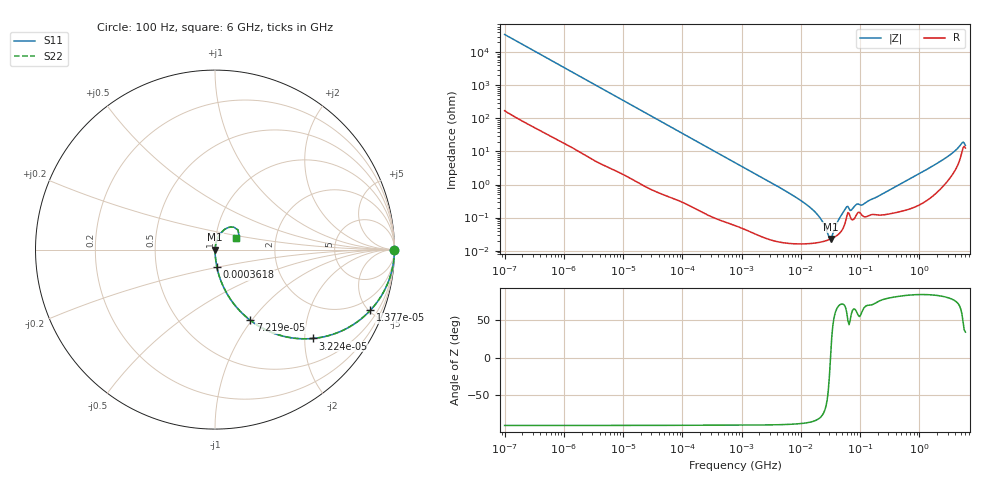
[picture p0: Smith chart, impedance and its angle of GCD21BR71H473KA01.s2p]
!Murata Part Number: GCD21BR71H473KA01
!These Parameters are Measured in Series Mode Connection
!Data Generated on Jan 08, 2026
!  o--ll--o
!Port1  Port2
!  o------o
!Operation Temp=25[degC], DC Bias Voltage=0[V]
!Freq. Start=100[Hz] Stop=6[GHz] 401[Steps]
# Hz S RI R 50
!Freq.(Hz) S11(Real) S11(Imag) S21(Real) S21(Imag) S12(Real) S12(Imag) S22(Real) S22(Imag)
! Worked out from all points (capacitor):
!   401 points, 100 Hz to 6 GHz, reference 50 ohm
!   read as one part in series: C = 45.8 nF near 109 Hz
!   lowest |Z| = 22.4 mohm at 31.85 MHz (marker M1)
!   series resonance near 31.67 MHz, so ESL is about 550 pH
!   S11 on the Smith chart (normalised r, x): 100 Hz: open; 13.77 kHz: 1.03, -5.12; 32.24 kHz: 1.01, -2.19; 72.19 kHz: 1.01, -0.98; 361.8 kHz: 1.00, -0.20; 6 GHz: 1.25, +0.17
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100  1 -0.00288  2.25e-05 0.00288  2.25e-05 0.00288  1 -0.00288
2008  0.9964 -0.0571  0.00356 0.0571  0.00356 0.0571  0.9964 -0.0571
13772  0.8662 -0.3376  0.1338 0.3376  0.1338 0.3376  0.8662 -0.3376
32244  0.5457 -0.4949  0.4543 0.4949  0.4543 0.4949  0.5457 -0.4949
40335  0.4352 -0.4926  0.5648 0.4926  0.5648 0.4926  0.4352 -0.4926
72189  0.1962 -0.3934  0.8038 0.3934  0.8038 0.3934  0.1962 -0.3934
141303  0.0615 -0.2359  0.9385 0.2359  0.9385 0.2359  0.0615 -0.2359
361830  0.0106 -0.0977  0.9894 0.0977  0.9894 0.0977  0.0106 -0.0977
774597  0.00271 -0.0462  0.9973 0.0462  0.9973 0.0462  0.00271 -0.0462
6644369  0.000191 -0.00523  0.9998 0.00523  0.9998 0.00523  0.000191 -0.00523
1.555665e7  0.000169 -0.00178  0.9998 0.00178  0.9998 0.00178  0.000169 -0.00178
2.128304e7  0.000181 -0.000947  0.9998 0.000947  0.9998 0.000947  0.000181 -0.000947
2.911731e7  0.00021 -0.000198  0.9998 0.000198  0.9998 0.000198  0.00021 -0.000198
3.184506e7  0.000224 1.3e-05  0.9998 -1.3e-05  0.9998 -1.3e-05  0.000224 1.3e-05
5.699437e7  0.000771 0.00174  0.9992 -0.00174  0.9992 -0.00174  0.000771 0.00174
7.129496e7  0.000893 0.00142  0.9991 -0.00142  0.9991 -0.00142  0.000893 0.00142
8.918374e7  0.00131 0.0022  0.9987 -0.0022  0.9987 -0.0022  0.00131 0.0022
1.115611e8  0.00111 0.0022  0.9989 -0.0022  0.9989 -0.0022  0.00111 0.0022
3.124326e8  0.00133 0.00664  0.9987 -0.00664  0.9987 -0.00664  0.00133 0.00664
2.34314e9  0.0102 0.0507  0.9898 -0.0507  0.9898 -0.0507  0.0102 0.0507
5.016141e9  0.0832 0.1255  0.9168 -0.1255  0.9168 -0.1255  0.0832 0.1255
6e9  0.118 0.0669  0.882 -0.0669  0.882 -0.0669  0.118 0.0669
